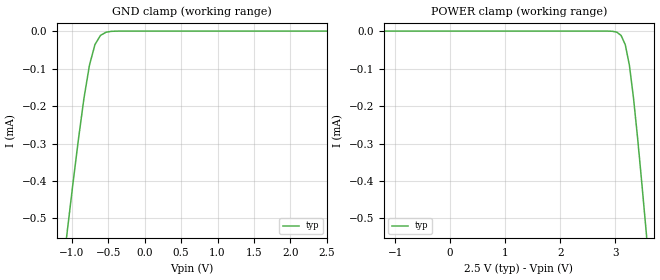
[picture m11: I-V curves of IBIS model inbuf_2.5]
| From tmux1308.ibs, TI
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| inbuf_2.5
[Model]   inbuf_2.5
Model_type   Input
Vinl = 0.7
Vinh = 1.1
|   typ   min   max
C_comp   4.014581e-14   NA   NA
[Voltage Range]   2.5   NA   NA
[Temperature Range]   27   NA   NA
[Power Clamp Reference]   2.5   NA   NA
[GND Clamp Reference]   0   NA   NA
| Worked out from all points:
|   GND clamp passes 1 mA (typ) near -1.33 V on its own axis
[GND Clamp]
|   Voltage   I(typ)   I(min)   I(max)
-5V       -7.717mA   NA         NA
-1.061V   -532.2uA   NA         NA
-984.8mV  -408.2uA   NA         NA
-909.1mV  -289.4uA   NA         NA
-833.3mV  -180uA     NA         NA
-757.6mV  -91.08uA   NA         NA
-681.8mV  -35.94uA   NA         NA
-606.1mV  -11.52uA   NA         NA
-530.3mV  -3.024uA   NA         NA
-378.8mV  -96.17nA   NA         NA
2.5V      36.2pA     NA         NA
[POWER Clamp]
|   Voltage   I(typ)   I(min)   I(max)
-2.5V     348pA      NA         NA
2.803V    -11.97nA   NA         NA
3.03V     -3.024uA   NA         NA
3.106V    -11.52uA   NA         NA
3.182V    -35.94uA   NA         NA
3.258V    -91.08uA   NA         NA
3.333V    -180uA     NA         NA
3.409V    -289.4uA   NA         NA
3.485V    -408.2uA   NA         NA
3.561V    -532.2uA   NA         NA
5V        -3.096mA   NA         NA
